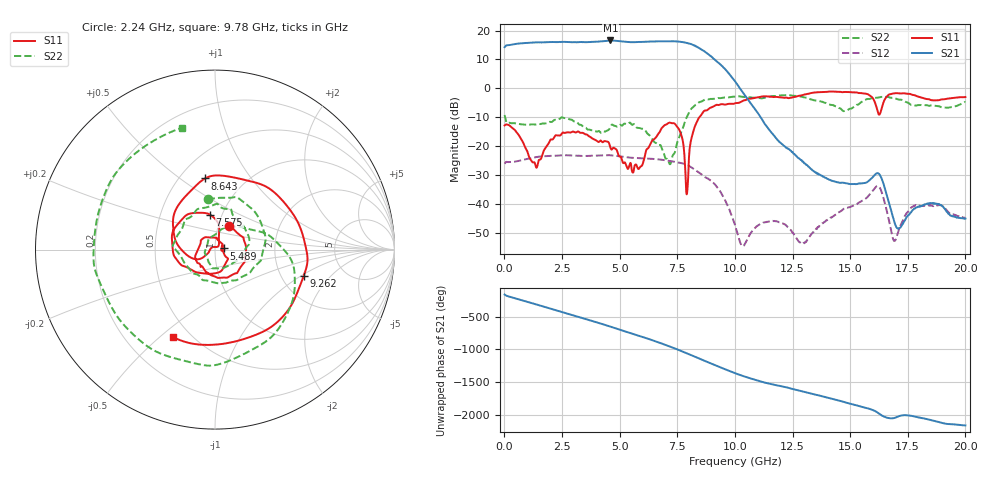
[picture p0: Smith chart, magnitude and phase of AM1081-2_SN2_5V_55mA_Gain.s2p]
!Agilent Technologies,E8364B,MY43040894,A.07.50.67
!Agilent E8364B: A.07.50.67
!Date: Wednesday, June 23, 2021 07:36:21
!Correction: S11(Full 2 Port(1,2))
!S21(Full 2 Port(1,2))
!S12(Full 2 Port(1,2))
!S22(Full 2 Port(1,2))
!S2P File: Measurements: S11, S21, S12, S22:
# Hz S  dB  R 50
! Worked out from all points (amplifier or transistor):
!   3201 points, 10 MHz to 20 GHz, reference 50 ohm
!   highest |S21| = 16.6 dB at 4.601 GHz (marker M1)
!   |S21| within 3 dB of that: start of sweep to 8.521 GHz
!   unconditionally stable (mu >= 1): start of sweep to end of sweep
!   at 3.34 GHz: K = 1.24, MAG = 16.7 dB, |S12| = -23.3 dB
!   at 10.01 GHz: K = 29.71, MAG = 7.1 dB, |S12| = -47.3 dB
!   at 20 GHz: K = 5121.32, MAG = -40.2 dB, |S12| = -44.8 dB
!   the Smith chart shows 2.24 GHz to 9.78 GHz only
!   S11 on the Smith chart (normalised r, x): 2.24 GHz: 1.13, +0.31; 5.489 GHz: 1.10, +0.01; 7.575 GHz: 0.88, +0.36; 8.643 GHz: 0.66, +0.62; 9.262 GHz: 2.64, -1.06; 9.78 GHz: 0.40, -0.55
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1e7  -12.83 -167.2  14.25 -166.7  -26.05 15.2  -9.21 60.2
1.028241e9  -22.62 85.0  15.74 79.6  -24.32 -81.2  -12.57 -138.7
1.671669e9  -22.39 110.4  15.91 13.5  -23.49 -141.2  -12.16 155.5
2.240134e9  -16.20 59.4  15.99 -45.4  -23.27 164.5  -10.92 98.2
2.758625e9  -15.21 2.8  16.02 -99.4  -23.14 113.1  -10.54 31.0
3.345831e9  -15.38 -62.4  16.04 -160.1  -23.34 55.9  -12.73 -35.2
3.889309e9  -17.59 -113.5  16.11 143.7  -23.27 3.7  -14.69 -90.0
4.601453e9  -20.54 178.3  16.56 66.0  -23.15 -69.6  -13.34 -178.6
5.038734e9  -23.57 81.9  16.27 15.8  -23.58 -115.1  -12.62 133.2
5.488509e9  -26.11 7.4  15.97 -33.3  -23.98 -160.6  -12.17 85.0
6.081962e9  -23.84 -31.2  16.10 -99.9  -24.25 137.2  -14.23 10.1
6.675416e9  -15.72 -129.4  16.25 -171.1  -24.55 69.9  -19.49 -80.7
7.200153e9  -11.88 152.2  16.30 122.2  -25.17 6.5  -26.18 153.7
7.574966e9  -14.12 98.0  16.16 71.3  -25.69 -41.3  -17.12 62.2
8.068469e9  -19.13 -150.7  15.41 0.4  -27.11 -110.2  -7.49 -6.6
8.643181e9  -7.96 98.0  13.04 -85.8  -30.30 174.0  -4.13 -81.7
9.261622e9  -5.76 -16.6  8.99 -174.5  -34.60 86.6  -3.36 -171.8
9.780112e9  -5.33 -115.7  4.74 110.9  -42.31 8.3  -3.06 105.2
1.0005e10  -5.15 -158.8  2.46 80.3  -47.28 -31.0  -2.90 72.5
1.334083e10  -1.59 179.0  -28.12 126.7  -50.20 92.1  -3.90 12.7
1.667042e10  -2.22 7.3  -39.12 119.2  -45.16 116.7  -3.03 -73.5
2e10  -3.00 116.7  -45.03 7.1  -44.76 3.5  -4.75 -132.1
